(* Logix 5000 AddOnInstructionDefinition export Banner_S15C_MGP_PD_v2; software revision 32.00 *)

TYPE Banner_S15C_MGP_Data_Set_0 :
STRUCT
   Latitude : REAL;
   Longitude : REAL;
   Altitude : REAL;
   UTC_Time : DINT;   // Hr:Min:Sec in UTC
   Date : DINT;   // Day/Month/Year
   Signal_Quality : DINT;
   Num_Satellites : INT;   // Number of Satellites being tracked
   Time : DINT;   // Time in seconds since the last DGPS update
   Fix_2d_3d : INT;
END_STRUCT
END_TYPE

TYPE Banner_S15C_MGP_Data_Set_1 :
STRUCT
   PDOP : REAL;   // Position Dilution of Precision
   HDOP : REAL;   // Horizontal Dilution of Precision
   VDOP : REAL;   // Vertical Dilution of Precision
   Speed : REAL;
   Direction : REAL;
END_STRUCT
END_TYPE

TYPE Banner_S15C_MGP_Data_Set_2 :
STRUCT
   Serial_Num : DINT;
   Model_Num : DINT;
   Production_Date : DINT;
   RF_FW_Part_Num : DINT;
   RF_FW_Ver_Major : INT;
   RF_FW_Ver_Minor : INT;
   RF_FW_Version_Eng : DINT;
   RF_EEPROM_Part_Num : DINT;
   RF_EEPROM_Ver_Major : INT;
   RF_EEPROM_Ver_Minor : INT;
END_STRUCT
END_TYPE

TYPE Banner_S15C_MGP_PDIO_v2 :   // UDT with all of the variables needed to control an IO-Link S15C MGP.
STRUCT
   Read_Data_Set : SINT;   // 0 = VT English units, 1 = Metric units, 2 = Sensor Information
   Read_Status : SINT;   // 0 = failed, 1 = success
   Counter_Value : INT;
   Data_Set_0 : Banner_S15C_MGP_Data_Set_0;
   Data_Set_1 : Banner_S15C_MGP_Data_Set_1;
   Data_Set_2 : Banner_S15C_MGP_Data_Set_2;   // Sensor Information Data Set
   DTI : SINT[32];   // Array with Raw Process data being transferred into AOI.
   Write_Data_Set : SINT;   // Set which Data Set should be gathered via the S15C.
END_STRUCT
END_TYPE

ADD_ON_INSTRUCTION Banner_S15C_MGP_PD_v2   (* revision 2.0, vendor Banner Engineering *)
// AOI that used with the S15C MEZ sensor.
VAR_IN_OUT
   Process_Data : Banner_S15C_MGP_PDIO_v2; {required}
END_VAR
VAR_INPUT
   Byte_Swap : BOOL; {required}
END_VAR
VAR
   Temp : INT[16]; {access None}
   W_Index : SINT; {access None}
   DT_Index : SINT; {access None}
   Data_Update : BOOL; {access None}
   TempConvert : DINT[6]; {access None}
END_VAR

ROUTINE Logic   (* ladder *)
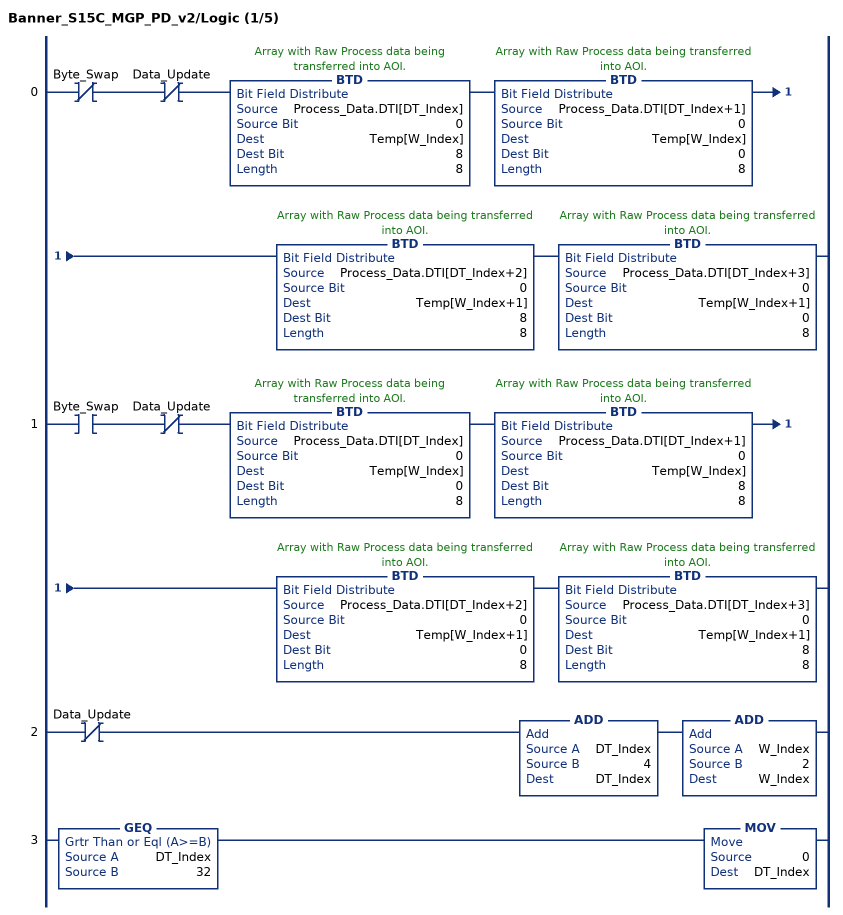
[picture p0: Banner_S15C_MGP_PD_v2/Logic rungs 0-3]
   0: XIO(Byte_Swap)XIO(Data_Update)BTD(Process_Data.DTI[DT_Index],0,Temp[W_Index],8,8)BTD(Process_Data.DTI[DT_Index+1],0,Temp[W_Index],0,8)BTD(Process_Data.DTI[DT_Index+2],0,Temp[W_Index+1],8,8)BTD(Process_Data.DTI[DT_Index+3],0,Temp[W_Index+1],0,8);
   1: XIC(Byte_Swap)XIO(Data_Update)BTD(Process_Data.DTI[DT_Index],0,Temp[W_Index],0,8)BTD(Process_Data.DTI[DT_Index+1],0,Temp[W_Index],8,8)BTD(Process_Data.DTI[DT_Index+2],0,Temp[W_Index+1],0,8)BTD(Process_Data.DTI[DT_Index+3],0,Temp[W_Index+1],8,8);
   2: XIO(Data_Update)ADD(DT_Index,4,DT_Index)ADD(W_Index,2,W_Index);
   3: GEQ(DT_Index,32)MOV(0,DT_Index);
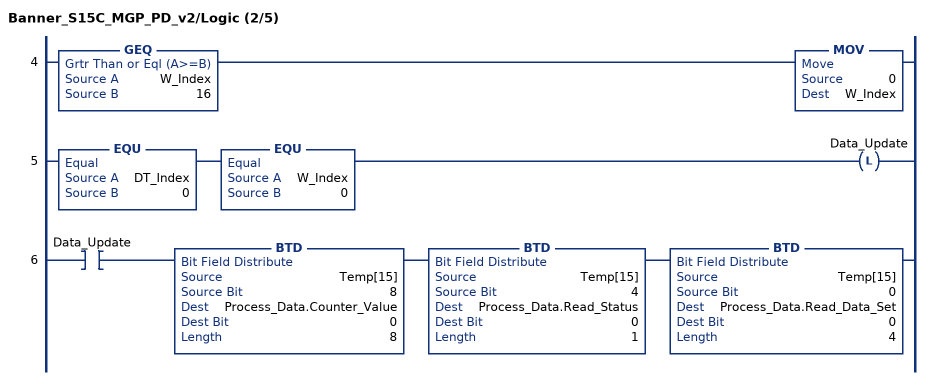
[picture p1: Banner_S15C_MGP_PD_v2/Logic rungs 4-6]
   4: GEQ(W_Index,16)MOV(0,W_Index);
   5: EQU(DT_Index,0)EQU(W_Index,0)OTL(Data_Update);
   6: XIC(Data_Update)BTD(Temp[15],8,Process_Data.Counter_Value,0,8)BTD(Temp[15],4,Process_Data.Read_Status,0,1)BTD(Temp[15],0,Process_Data.Read_Data_Set,0,4);
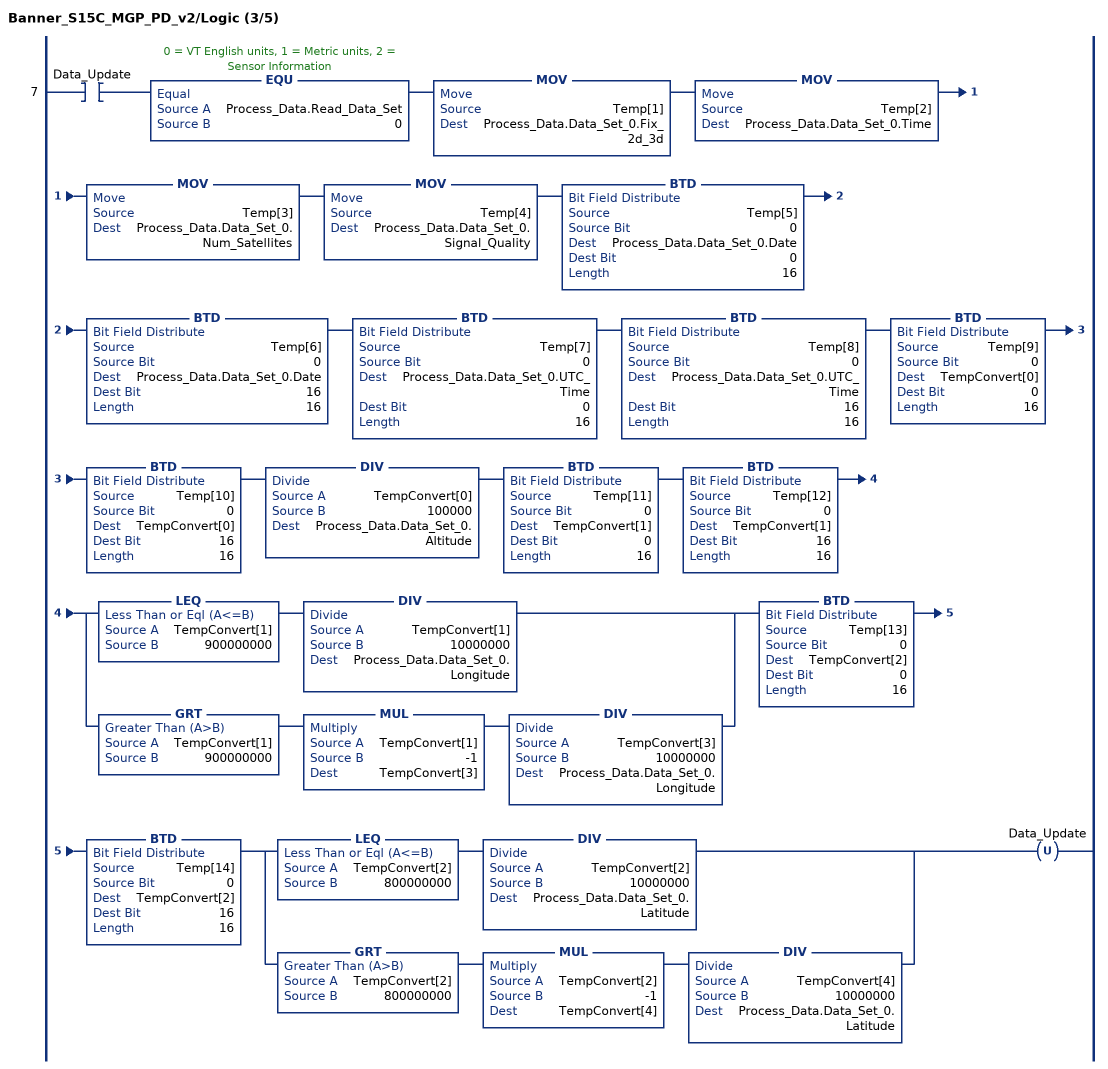
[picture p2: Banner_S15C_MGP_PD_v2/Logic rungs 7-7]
   7: XIC(Data_Update)EQU(Process_Data.Read_Data_Set,0)MOV(Temp[1],Process_Data.Data_Set_0.Fix_2d_3d)MOV(Temp[2],Process_Data.Data_Set_0.Time)MOV(Temp[3],Process_Data.Data_Set_0.Num_Satellites)MOV(Temp[4],Process_Data.Data_Set_0.Signal_Quality)BTD(Temp[5],0,Process_Data.Data_Set_0.Date,0,16)BTD(Temp[6],0,Process_Data.Data_Set_0.Date,16,16)BTD(Temp[7],0,Process_Data.Data_Set_0.UTC_Time,0,16)BTD(Temp[8],0,Process_Data.Data_Set_0.UTC_Time,16,16)BTD(Temp[9],0,TempConvert[0],0,16)BTD(Temp[10],0,TempConvert[0],16,16)DIV(TempConvert[0],100000,Process_Data.Data_Set_0.Altitude)BTD(Temp[11],0,TempConvert[1],0,16)BTD(Temp[12],0,TempConvert[1],16,16)[LEQ(TempConvert[1],900000000) DIV(TempConvert[1],10000000,Process_Data.Data_Set_0.Longitude) ,GRT(TempConvert[1],900000000) MUL(TempConvert[1],-1,TempConvert[3]) DIV(TempConvert[3],10000000,Process_Data.Data_Set_0.Longitude) ]BTD(Temp[13],0,TempConvert[2],0,16)BTD(Temp[14],0,TempConvert[2],16,16)[LEQ(TempConvert[2],800000000) DIV(TempConvert[2],10000000,Process_Data.Data_Set_0.Latitude) ,GRT(TempConvert[2],800000000) MUL(TempConvert[2],-1,TempConvert[4]) DIV(TempConvert[4],10000000,Process_Data.Data_Set_0.Latitude) ]OTU(Data_Update);
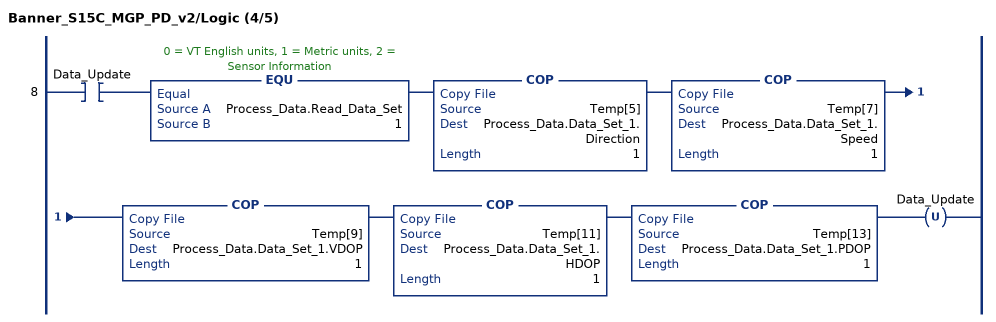
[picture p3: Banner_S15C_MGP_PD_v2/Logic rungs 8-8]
   8: XIC(Data_Update)EQU(Process_Data.Read_Data_Set,1)COP(Temp[5],Process_Data.Data_Set_1.Direction,1)COP(Temp[7],Process_Data.Data_Set_1.Speed,1)COP(Temp[9],Process_Data.Data_Set_1.VDOP,1)COP(Temp[11],Process_Data.Data_Set_1.HDOP,1)COP(Temp[13],Process_Data.Data_Set_1.PDOP,1)OTU(Data_Update);
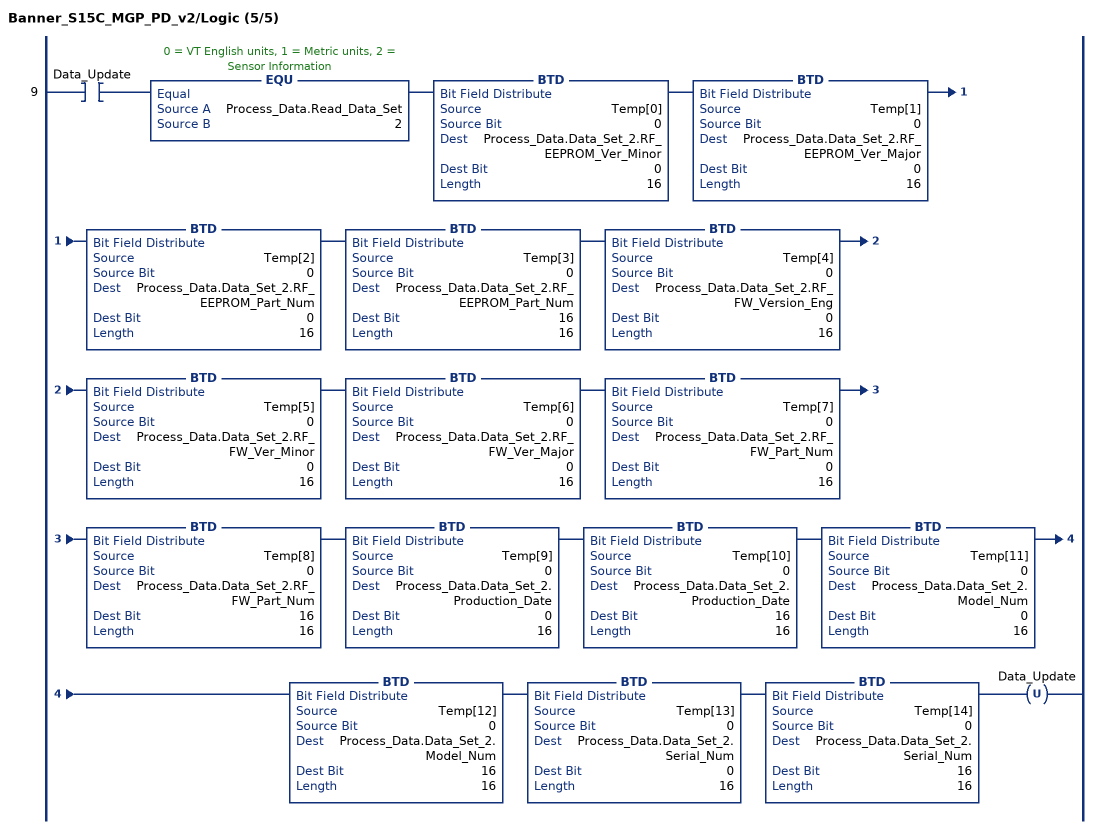
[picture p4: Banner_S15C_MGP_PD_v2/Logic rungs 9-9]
   9: XIC(Data_Update)EQU(Process_Data.Read_Data_Set,2)BTD(Temp[0],0,Process_Data.Data_Set_2.RF_EEPROM_Ver_Minor,0,16)BTD(Temp[1],0,Process_Data.Data_Set_2.RF_EEPROM_Ver_Major,0,16)BTD(Temp[2],0,Process_Data.Data_Set_2.RF_EEPROM_Part_Num,0,16)BTD(Temp[3],0,Process_Data.Data_Set_2.RF_EEPROM_Part_Num,16,16)BTD(Temp[4],0,Process_Data.Data_Set_2.RF_FW_Version_Eng,0,16)BTD(Temp[5],0,Process_Data.Data_Set_2.RF_FW_Ver_Minor,0,16)BTD(Temp[6],0,Process_Data.Data_Set_2.RF_FW_Ver_Major,0,16)BTD(Temp[7],0,Process_Data.Data_Set_2.RF_FW_Part_Num,0,16)BTD(Temp[8],0,Process_Data.Data_Set_2.RF_FW_Part_Num,16,16)BTD(Temp[9],0,Process_Data.Data_Set_2.Production_Date,0,16)BTD(Temp[10],0,Process_Data.Data_Set_2.Production_Date,16,16)BTD(Temp[11],0,Process_Data.Data_Set_2.Model_Num,0,16)BTD(Temp[12],0,Process_Data.Data_Set_2.Model_Num,16,16)BTD(Temp[13],0,Process_Data.Data_Set_2.Serial_Num,0,16)BTD(Temp[14],0,Process_Data.Data_Set_2.Serial_Num,16,16)OTU(Data_Update);
END_ROUTINE
END_ADD_ON_INSTRUCTION
